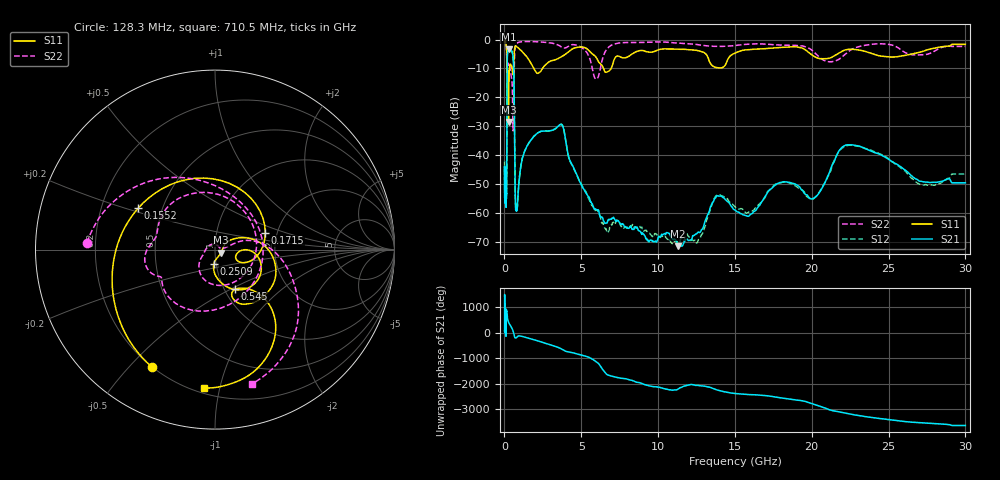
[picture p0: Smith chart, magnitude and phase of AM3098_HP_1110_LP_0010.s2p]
! Date/Time: Thu, Feb 28, 2019 8:46 AM
! Network Analyzer: Agilent Technologies E8364B Rev: A.07.50.67
! Sweep from 0.010 to 30.000 GHz, 1601 Points, Sweep Type: LOG
! Power Supply: 5.023 V, 0.002 A
# Hz S DB R 50
!freq MagS11 AngS11 MagS21 AngS21 MagS12 AngS12 MagS22 AngS22
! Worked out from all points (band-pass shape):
!   1601 points, 10 MHz to 30 GHz, reference 50 ohm
!   highest |S21| = -3.37 dB at 288.7 MHz (marker M1); lowest = -71.6 dB at 11.31 GHz (marker M2)
!   |S21| within 3 dB of the highest: 183.3 MHz to 567.6 MHz (384.2 MHz wide, 102 % of centre)
!   lowest |S11| = -28.6 dB at 263.8 MHz (marker M3), VSWR 1.08, Z = 53.4 - j1.77 ohm
!   |S11| at or under -10 dB: 170 MHz to 322.5 MHz (152.4 MHz wide, 61.9 % of centre); 1.909 GHz to 2.474 GHz (565.6 MHz wide, 25.8 % of centre); 6.454 GHz to 6.94 GHz (485.6 MHz wide, 7.25 % of centre)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
!   |S22| runs from -31.6 to -0.5 dB; largest |S21 - S12| = 0.013
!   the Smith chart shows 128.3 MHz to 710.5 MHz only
!   S11 on the Smith chart (normalised r, x): 128.3 MHz: 0.20, -0.58; 155.2 MHz: 0.37, +0.22; 171.5 MHz: 1.73, +0.36; 250.9 MHz: 0.97, -0.16; 545 MHz: 1.12, -0.53; 710.5 MHz: 0.23, -0.89
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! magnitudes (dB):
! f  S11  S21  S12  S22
! 10 MHz  -0.4  -44.1  -42.1  -0.6
! 38.04 MHz  -0.3  -50.1  -50.3  -0.6
! 128.3 MHz  -2.6  -53.9  -53.6  -2.9
! 144.7 MHz  -4.3  -49.5  -50.2  -5.7
! 155.2 MHz  -6.3  -34.4  -34.1  -10.5
! 171.5 MHz  -10.6  -11.5  -11.5  -8.7
! 250.9 MHz  -22.0  -3.6  -3.5  -9.1
! 263.8 MHz  -28.6  -3.4  -3.4  -9.4
! 288.7 MHz  -15.6  -3.4  -3.3  -9.4
! 485.7 MHz  -9.8  -4.1  -4.1  -14.1
! 545 MHz  -12.1  -5.3  -5.3  -28.7
! 550.5 MHz  -12.1  -5.5  -5.5  -29.8
! 617.6 MHz  -6.4  -13.4  -13.4  -13.7
! 710.5 MHz  -2.2  -55.7  -55.6  -2.2
! 2.084 GHz  -11.5  -32.7  -32.7  -0.7
! 3.723 GHz  -5.9  -29.4  -29.4  -2.6
! 5.989 GHz  -6.3  -59.0  -59.0  -13.7
! 7.926 GHz  -6.2  -65.0  -65.2  -1.0
! 11.31 GHz  -3.3  -71.6  -69.9  -1.2
! 20.1 GHz  -5.6  -55.0  -55.2  -4.1
! 22.56 GHz  -3.3  -36.4  -36.6  -3.5
! 30 GHz  -1.6  -49.6  -46.6  -2.3
